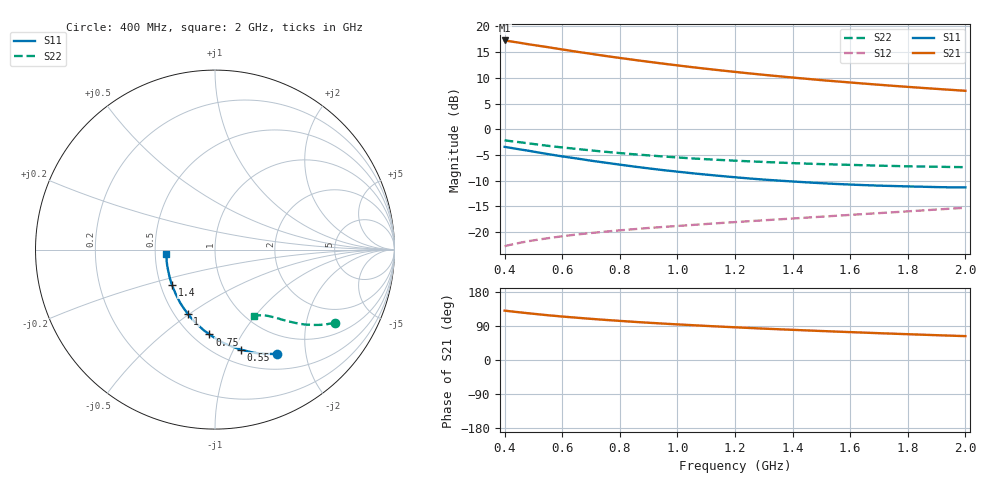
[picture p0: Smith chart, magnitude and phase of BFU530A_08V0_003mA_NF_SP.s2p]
! Filename:  P:\Prog\Test\Noise\ATS_data\Testdata_Net\06 Compressed Noise after Statistics\BFU530A_APG2013_33_A05_08p0V_003mA_NF_CM01_D.sf
! Date/Time: Tue 16/Apr/2013 15:10:57
! BFU530A_APG2013_33_A05_08p0V_1to25mA_NF_CM01_Bias3_R.sf
! Noise Parameter Data File
! BFU530A_APG2013_33_A05_08p0V_1to25mA_NF_CM01
! Date/time: Fri Apr 12 16:45:05 2013
! VAR V_out= 8.001000
! VAR I_out= 3.000000
! VAR V_in= 0.805100
! VAR I_in= 0.030410
! Device data file deembeded for feedlines and parallel
! Original file: \06 Compressed Noise after Statistics\BFU530A_APG2013_33_A05_08p0V_003mA_NF_CM01_R.sf
! Feed-files: PR017V01_150413_Feed1.s2p, PR017V01_150413_Feed2.s2p
! Parallel-file: PR017V01_150413_Par.s2p
# MHz S MA R 50
!  Freq-MHz  S11-mag  S11-arg  S21-mag  S21-arg  S12-mag  S12-arg  S22-mag  S22-arg
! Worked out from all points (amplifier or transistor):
!   37 points, 400 MHz to 2 GHz, reference 50 ohm
!   highest |S21| = 17.3 dB at 400 MHz (marker M1)
!   |S21| within 3 dB of that: start of sweep to 748.2 MHz
!   unconditionally stable (mu >= 1): 1.866 GHz to end of sweep
!   at 500 MHz: K = 0.44, MSG = 19.0 dB, |S12| = -21.6 dB
!   at 1.1 GHz: K = 0.80, MSG = 15.1 dB, |S12| = -18.4 dB
!   at 2 GHz: K = 1.01, MAG = 10.7 dB, |S12| = -15.2 dB
!   lowest NFmin = 0.48 dB at 420 MHz
!   S11 on the Smith chart (normalised r, x): 400 MHz: 0.71, -1.52; 550 MHz: 0.64, -1.06; 750 MHz: 0.60, -0.74; 1 GHz: 0.58, -0.49; 1.4 GHz: 0.57, -0.25; 2 GHz: 0.57, -0.03
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400  0.6754 -59.1  7.315 130.4  0.07309 60.5  0.7815 -31.3
420  0.6613 -61.5  7.173 128.5  0.07534 59.6  0.7685 -32.3
440  0.6469 -63.8  7.031 126.8  0.07747 58.9  0.7562 -33.2
480  0.6211 -68.2  6.736 123.5  0.08139 57.5  0.7318 -34.9
550  0.5747 -75.7  6.296 118.1  0.08732 55.6  0.6914 -37.4
600  0.5457 -80.5  5.983 114.7  0.09124 54.6  0.6667 -38.9
650  0.5209 -85.0  5.685 111.6  0.0949 53.7  0.6449 -40.2
700  0.4956 -89.5  5.426 108.6  0.09808 53.0  0.6237 -41.4
750  0.474 -93.7  5.169 105.8  0.1012 52.5  0.6047 -42.5
800  0.4536 -97.9  4.947 103.2  0.1042 52.2  0.5878 -43.4
850  0.4343 -102.0  4.734 100.7  0.107 51.9  0.5718 -44.3
900  0.4171 -105.9  4.538 98.3  0.1099 51.7  0.5583 -45.2
950  0.4015 -109.6  4.356 96.1  0.1123 51.7  0.5446 -46.0
1000  0.3876 -113.2  4.186 94.0  0.1149 51.7  0.5331 -46.7
1100  0.3627 -120.4  3.881 90.0  0.1201 51.9  0.5123 -48.0
1200  0.3419 -127.2  3.618 86.3  0.1253 52.2  0.4956 -49.3
1300  0.3245 -133.7  3.39 82.8  0.1305 52.6  0.4817 -50.6
1400  0.3111 -140.3  3.188 79.6  0.1358 53.2  0.4693 -51.8
1500  0.2994 -146.5  3.009 76.5  0.1413 53.7  0.4592 -53.1
1650  0.2867 -155.4  2.782 72.2  0.1502 54.6  0.4473 -55.0
1750  0.281 -161.2  2.648 69.4  0.1562 55.2  0.4403 -56.3
2000  0.2726 -174.6  2.37 63.0  0.1728 56.5  0.4287 -60.0
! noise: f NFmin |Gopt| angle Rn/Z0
400  0.5695  0.3326  23.52  0.1532
460  0.556  0.3367  26.45  0.1504
600  0.6281  0.3456  31.48  0.1648
800  0.6359  0.3263  53.02  0.1276
1000  0.6556  0.3262  64.78  0.1197
1200  0.7248  0.3174  78.19  0.1134
1400  0.7478  0.2959  96.68  0.0986
1600  0.8011  0.2682  112  0.0881
1800  0.7808  0.302  128.4  0.0694
2000  0.7631  0.2433  144  0.0822
